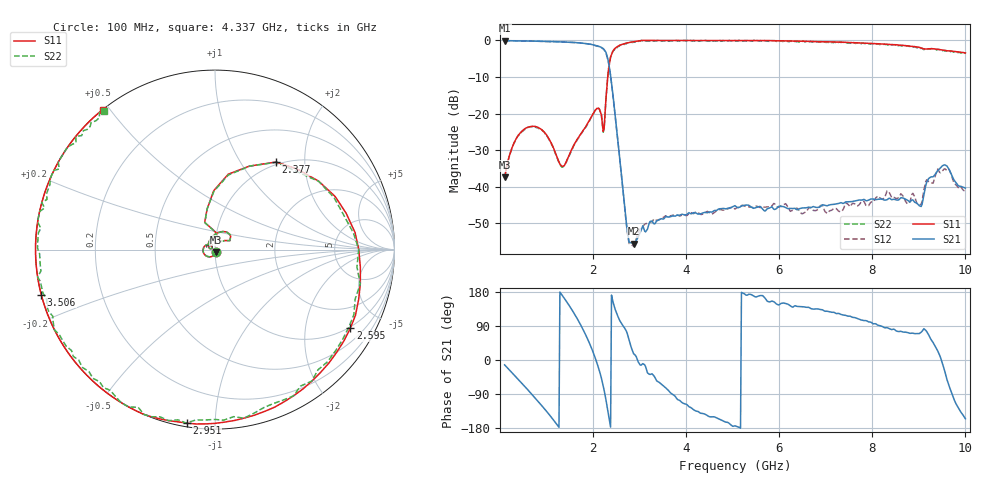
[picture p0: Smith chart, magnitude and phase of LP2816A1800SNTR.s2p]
!	AVX	THIN	FILM	OPERATION
!	LP2816S	High	Performance	Low	Pass	Filters
!	P/N	LP2816A1800SNTR
!	Created	22	November	2016
!Instrument:	"HEWLETT PACKARD,8720ES,US39172150,7.62 "
#	MHz	S	dB	R	50
!	Frq	S11(dB)	S11(deg)	S21(dB)	S21(deg)	S12(dB)	S12(deg)	S22(dB)	S22(deg)
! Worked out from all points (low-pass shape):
!   501 points, 100 MHz to 10 GHz, reference 50 ohm
!   highest |S21| = -0.03 dB at 100 MHz (marker M1); lowest = -55.5 dB at 2.872 GHz (marker M2)
!   |S21| within 3 dB of the highest: start of sweep to 2.266 GHz
!   lowest |S11| = -37.5 dB at 100 MHz (marker M3), VSWR 1.03, Z = 50.4 - j1.27 ohm
!   |S11| at or under -10 dB: start of sweep to 2.315 GHz
!   |S22| runs from -37.5 to 0.0 dB; largest |S21 - S12| = 0.02
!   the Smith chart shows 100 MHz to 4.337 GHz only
!   S11 on the Smith chart (normalised r, x): 100 MHz: 1.01, -0.03; 2.377 GHz: 0.96, +1.45; 2.595 GHz: 0.95, -3.48; 2.951 GHz: 0.02, -0.85; 3.506 GHz: 0.00, -0.13; 4.337 GHz: 0.00, +0.48
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100  -37.45 -69.8  -0.03 -12.9  -0.05 -13.1  -37.45 -69.9
674.2  -23.50 -167.9  -0.18 -89.0  -0.17 -89.3  -23.60 -167.9
1208.8  -31.34 133.2  -0.34 -167.8  -0.37 -167.9  -31.34 133.1
1486  -31.36 169.6  -0.47 144.0  -0.47 143.8  -31.56 169.6
1763.2  -25.10 126.4  -0.73 85.8  -0.76 85.4  -25.20 126.2
2060.2  -18.89 61.4  -1.37 0.6  -1.42 -0.1  -18.89 61.4
2238.4  -23.99 70.0  -2.50 -79.7  -2.60 -80.9  -24.19 69.8
2377  -4.51 55.1  -9.54 -177.1  -9.65 -177.9  -4.51 54.9
2476  -2.09 7.0  -20.52 133.4  -20.72 133.8  -2.19 6.8
2594.8  -1.19 -30.1  -34.71 99.7  -34.98 99.6  -1.29 -30.2
2753.2  -0.62 -65.5  -53.38 61.9  -53.79 63.5  -0.72 -65.7
2872  -0.33 -86.9  -55.53 16.5  -56.23 13.2  -0.43 -87.1
2951.2  -0.18 -99.3  -54.16 1.4  -53.27 -0.8  -0.18 -99.5
3406.6  0.00 -155.7  -49.11 -57.8  -49.00 -55.4  -0.10 -155.7
3505.6  0.00 -165.5  -48.83 -67.6  -48.38 -65.4  -0.10 -165.7
4337.2  0.00 128.8  -47.26 -140.9  -47.53 -142.8  -0.10 128.6
5050  0.00 88.0  -45.16 -173.7  -46.09 -177.4  0.00 88.0
6713.2  -0.28 18.1  -45.51 134.7  -46.13 125.6  -0.48 18.1
8356.6  -1.08 -42.2  -43.16 83.3  -41.45 84.0  -1.08 -42.4
9029.8  -1.97 -72.2  -45.29 71.5  -44.87 72.9  -2.17 -72.5
9544.6  -2.68 -95.4  -34.03 -24.4  -35.11 -25.8  -2.78 -95.5
10000  -3.42 -120.9  -40.36 -155.1  -41.20 -146.3  -3.42 -120.9
